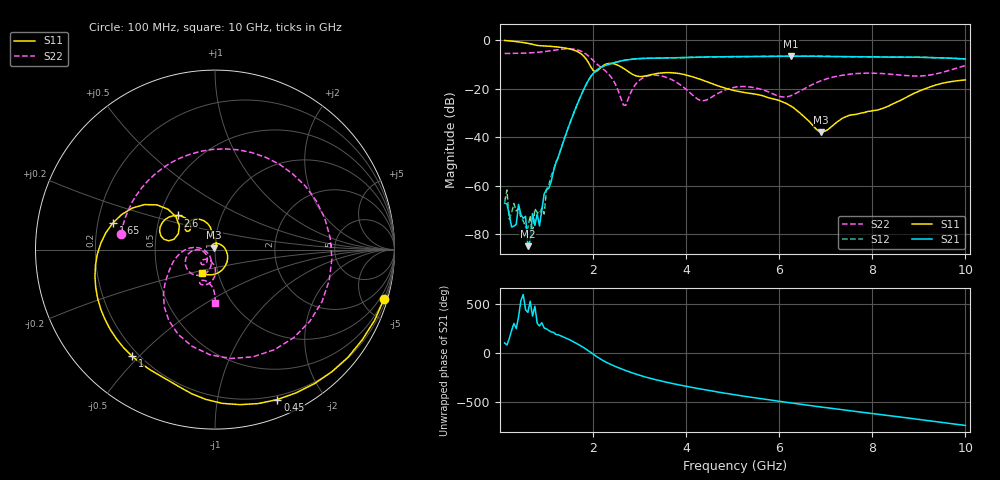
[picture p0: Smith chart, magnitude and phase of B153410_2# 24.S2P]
!  2-Port S-parameters saved by WinCal
! VAR MeasName=S-Parameters (CALIBRATED_DATA) read from VNA (N5245A)
! VAR MeasDate=2016-12-23 10:00:33
! VAR NAME=B153410_2# 24
! VAR FILENAME=B153410_2# 24.S2P
! VAR DATE=2016-12-23 10:00:33
! VAR PHYS_PORTS=1,2
# Hz S DB R 50
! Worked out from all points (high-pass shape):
!   199 points, 100 MHz to 10 GHz, reference 50 ohm
!   highest |S21| = -6.63 dB at 6.25 GHz (marker M1); lowest = -84.8 dB at 600 MHz (marker M2)
!   |S21| within 3 dB of the highest: 2.395 GHz to end of sweep
!   lowest |S11| = -37.9 dB at 6.9 GHz (marker M3), VSWR 1.03, Z = 49.5 + j1.15 ohm
!   |S11| at or under -10 dB: 1.922 GHz to 2.27 GHz (347.5 MHz wide, 16.6 % of centre); 2.484 GHz to end of sweep
!   |S22| runs from -26.9 to -3.6 dB; largest |S21 - S12| = 0.0026
!   S11 on the Smith chart (normalised r, x): 100 MHz: 0.47, -7.02; 450 MHz: 0.16, -1.49; 1 GHz: 0.17, -0.48; 1.65 GHz: 0.26, +0.12; 2.6 GHz: 0.62, +0.25; 10 GHz: 0.84, -0.23
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1e8  -0.16 -16.1  -67.12 99.2  -66.58 -104.2  -5.52 170.3
2.5e8  -0.41 -39.0  -76.92 -133.4  -71.14 27.3  -5.51 155.4
4.5e8  -0.87 -67.4  -71.87 171.5  -73.13 -119.0  -5.42 134.3
6e8  -1.33 -87.3  -84.84 51.5  -77.37 -113.5  -5.31 117.2
6.5e8  -1.55 -93.5  -82.47 164.8  -72.24 -144.4  -5.26 111.2
7e8  -1.80 -99.2  -71.40 13.6  -80.76 101.9  -5.21 104.8
7.5e8  -2.04 -104.3  -76.29 113.9  -69.37 -38.8  -5.14 98.3
8.5e8  -2.31 -113.5  -76.54 -87.3  -71.43 -124.2  -4.98 84.4
9.5e8  -2.42 -122.9  -63.32 -108.6  -71.63 -99.4  -4.76 69.4
1e9  -2.47 -127.8  -61.62 -117.1  -61.61 -124.0  -4.64 61.3
1.35e9  -3.13 -162.4  -42.44 162.5  -42.46 162.7  -3.70 -4.5
1.65e9  -4.62 165.3  -26.93 93.7  -26.92 93.8  -3.96 -70.5
1.75e9  -5.76 153.3  -22.45 66.4  -22.43 66.2  -4.63 -92.7
2.6e9  -11.00 137.6  -8.61 -162.8  -8.62 -163.0  -24.07 -179.6
3.4e9  -13.66 143.5  -7.44 79.0  -7.45 78.9  -14.55 -149.7
4.35e9  -16.47 105.7  -7.00 -12.6  -7.01 -12.8  -24.99 -151.4
5.05e9  -20.87 101.5  -6.81 -68.4  -6.84 -68.3  -19.40 -128.5
6.25e9  -27.14 79.9  -6.63 -151.0  -6.64 -151.0  -22.90 -105.5
6.7e9  -34.68 81.5  -6.65 179.8  -6.67 179.8  -18.39 -88.7
6.9e9  -37.90 114.4  -6.69 167.2  -6.72 167.2  -16.73 -90.3
8.35e9  -27.18 34.8  -7.00 80.4  -7.00 80.6  -13.98 -115.2
1e10  -16.43 -118.6  -7.80 -20.5  -7.81 -20.4  -10.47 -90.0
